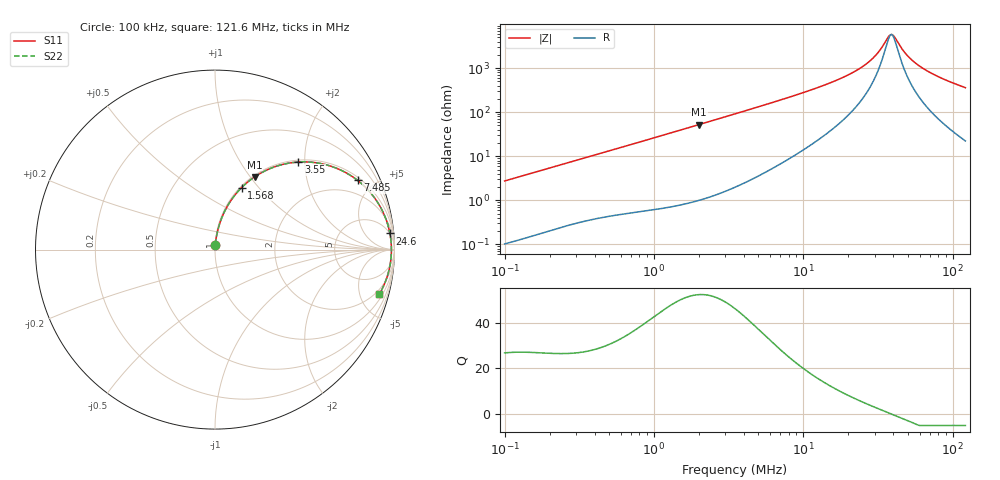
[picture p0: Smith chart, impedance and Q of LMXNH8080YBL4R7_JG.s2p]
! LMXNH8080YBL4R7_JG  S-PARAMETER MODEL  ( General Type )
! Model Generated by TAIYO YUDEN Corporation (http://www.ty-top.com)
! Version 1.0
! TAIYO YUDEN Control No. 191025NI43SB-FBB
! Copyright(c) 2019 TAIYO YUDEN CO.,LTD. All Rights Reserved.
! Product Description (link to TY-COMPAS)
! https://ds.yuden.co.jp/TYCOMPAS/or/detail?pn=LMXNH8080YBL4R7NJG&u=M
! Products Name : Inductors
! Characteristics :
!  Inductance : 4.7 uH , SRF(min) : 30 MHz , DC Resistance(max) : 0.0234 Ohm
!  Rated Current : Saturation :5400 mA , Temp Rise : 4100 mA
!  Case Size : 8.0 x 8.0 / 0.315 x 0.315 [mm/inch] , Thickness : 4.2 / 0.165 [mm/inch]
!  (Conditions: Temperature = 25 degC , DC Bias Current/Voltage = 0A / 0V)
! External Node Assignments :
!  1  o---GGG---o  2
! GND o---------o GND
! Frequency Range : 0.1MHz  -  121.638923MHz  [ 402 STEP ]
# MHz S RI R 50
! Freq[MHz].  S11 Real  S11 Imag  S21 Real  S21 Imag  S12 Real  S12 Imag  S22 Real  S22 Imag
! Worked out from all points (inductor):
!   401 points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, 100 kHz to 121.6 MHz, reference 50 ohm
!   read as one part in series: L = 4.36 uH near 103.6 kHz
!   highest Q = 52.2 at 2.011 MHz (marker M1), where L = 4.15 uH
!   self-resonance near 38.35 MHz
!   S11 on the Smith chart (normalised r, x): 100 kHz: 1.00, +0.06; 1.568 MHz: 1.02, +0.82; 3.55 MHz: 1.04, +1.86; 7.485 MHz: 1.15, +4.03; 24.6 MHz: 5, +21; 121.6 MHz: 1.45, -7.17
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0.1  0.00178 0.0274  0.9982 -0.0274  0.9982 -0.0274  0.00178 0.0274
0.328662  0.0108 0.0866  0.9892 -0.0866  0.9892 -0.0866  0.0108 0.0866
0.611918  0.0297 0.1554  0.9703 -0.1554  0.9703 -0.1554  0.0297 0.1554
1.080188  0.0788 0.2583  0.9212 -0.2583  0.9212 -0.2583  0.0788 0.2583
1.568432  0.1483 0.3456  0.8517 -0.3456  0.8517 -0.3456  0.1483 0.3456
2.011144  0.2203 0.405  0.7797 -0.405  0.7797 -0.405  0.2203 0.405
3.550168  0.4648 0.4879  0.5352 -0.4879  0.5352 -0.4879  0.4648 0.4879
4.974964  0.6299 0.4696  0.3701 -0.4696  0.3701 -0.4696  0.6299 0.4696
7.484824  0.7941 0.3859  0.2059 -0.3859  0.2059 -0.3859  0.7941 0.3859
11.46267  0.9008 0.2713  0.0992 -0.2713  0.0992 -0.2713  0.9008 0.2713
17.86911  0.9562 0.1596  0.0438 -0.1596  0.0438 -0.1596  0.9562 0.1596
24.59978  0.9746 0.0899  0.0254 -0.0899  0.0254 -0.0899  0.9746 0.0899
30.44272  0.9807 0.0472  0.0193 -0.0472  0.0193 -0.0472  0.9807 0.0472
32.68392  0.9818 0.0334  0.0182 -0.0334  0.0182 -0.0334  0.9818 0.0334
37.67347  0.983 0.00607  0.017 -0.00607  0.017 -0.00607  0.983 0.00607
39.03561  0.983 -0.000724  0.017 0.000724  0.017 0.000724  0.983 -0.000724
40.447  0.9829 -0.00752  0.0171 0.00752  0.0171 0.00752  0.9829 -0.00752
49.1729  0.9809 -0.0452  0.0191 0.0452  0.0191 0.0452  0.9809 -0.0452
53.73896  0.979 -0.0627  0.021 0.0627  0.021 0.0627  0.979 -0.0627
60.85244  0.9751 -0.0878  0.0249 0.0878  0.0249 0.0878  0.9751 -0.0878
82.29881  0.9585 -0.1533  0.0415 0.1533  0.0415 0.1533  0.9585 -0.1533
121.6389  0.9148 -0.2499  0.0852 0.2499  0.0852 0.2499  0.9148 -0.2499
